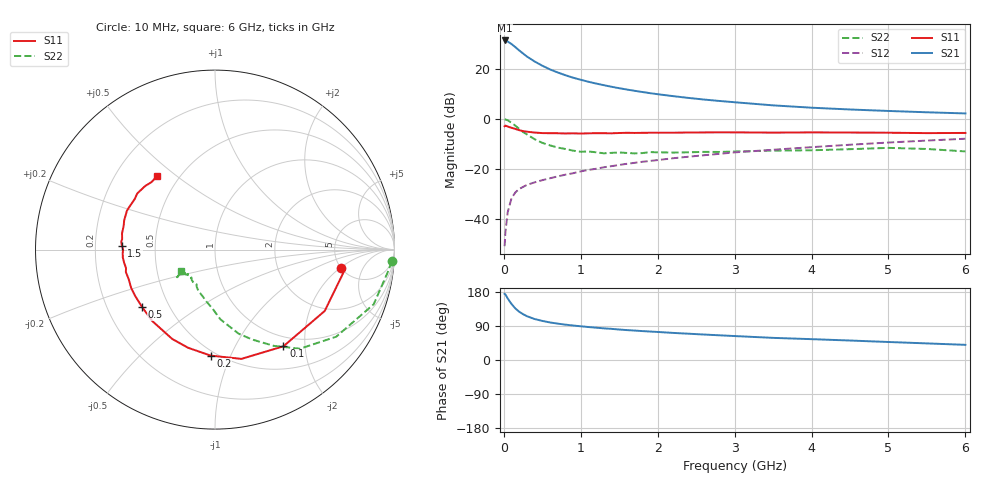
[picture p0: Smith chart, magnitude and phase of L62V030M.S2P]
!  INFINEON TECHNOLOGIES Small Signal Semiconductors
! BFR380L3 , Si-NPN RF-Transistor in TSLP-3-1
!  Vce=2 V,  Ic=30 mA
! Common Emitter S-Parameters:  07. March 2005
#  GHz  S  MA  R  50
! f  S11  S21  S12  S22
! GHz  Mag  Ang  Mag  Ang  Mag  Ang  Mag  Ang
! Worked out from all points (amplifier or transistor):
!   36 points, 10 MHz to 6 GHz, reference 50 ohm
!   highest |S21| = 31.4 dB at 10 MHz (marker M1)
!   |S21| within 3 dB of that: start of sweep to 162.2 MHz
!   unconditionally stable (mu >= 1): 1.783 GHz to 4.868 GHz
!   at 250 MHz: K = 0.41, MSG = 26.7 dB, |S12| = -27.3 dB
!   at 1.4 GHz: K = 0.97, MSG = 15.9 dB, |S12| = -19.0 dB
!   at 6 GHz: K = 0.98, MSG = 5.1 dB, |S12| = -8.0 dB
!   S11 on the Smith chart (normalised r, x): 10 MHz: 4.98, -2.07; 100 MHz: 0.84, -1.60; 200 MHz: 0.47, -0.85; 500 MHz: 0.35, -0.31; 1.5 GHz: 0.32, +0.02; 6 GHz: 0.38, +0.43
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0.01  0.709 -8.4  37.17 174.6  0.0028 82.3  0.9874 -3.8
0.02  0.7304 -9.2  36.77 173.1  0.0052 84.2  0.969 -7.8
0.05  0.7004 -29.2  35.46 162.5  0.0134 77.3  0.9352 -19.0
0.1  0.66 -54.7  31.53 147.7  0.0257 67.7  0.8317 -35.7
0.15  0.6264 -76.4  27.31 135.9  0.0335 59.3  0.7273 -49.4
0.2  0.5911 -92.3  23.44 127.3  0.0393 56.0  0.6283 -58.6
0.25  0.5672 -105.3  20.34 120.9  0.0431 53.2  0.5424 -67.5
0.3  0.552 -115.6  17.72 115.6  0.0474 51.8  0.4866 -74.3
0.4  0.5297 -131.4  14.08 108.1  0.0532 51.3  0.3895 -85.6
0.5  0.5172 -141.9  11.6 103.2  0.0589 52.6  0.3292 -92.4
0.6  0.5143 -149.9  9.764 99.1  0.0643 53.6  0.2934 -99.3
0.7  0.5136 -155.5  8.482 96.0  0.07 55.3  0.2655 -105.8
0.8  0.5083 -161.2  7.477 93.3  0.0759 56.9  0.2486 -111.8
0.9  0.512 -165.9  6.666 91.0  0.0811 57.9  0.2299 -116.4
1.1  0.5119 -172.0  5.524 87.0  0.0946 60.1  0.2212 -122.5
1.5  0.5192 177.6  4.105 80.4  0.1189 62.5  0.2112 -132.5
1.8  0.5232 171.6  3.445 76.3  0.1374 63.2  0.2054 -137.7
2.2  0.5259 165.3  2.846 71.5  0.1619 63.6  0.2105 -140.6
3.5  0.5285 147.8  1.859 58.4  0.2397 62.1  0.23 -145.4
4.5  0.5304 141.6  1.537 51.4  0.3023 60.5  0.2461 -144.8
5.5  0.5163 133.3  1.351 43.8  0.3664 56.8  0.2483 -144.6
6  0.521 128.3  1.281 40.0  0.3987 54.8  0.222 -147.4
